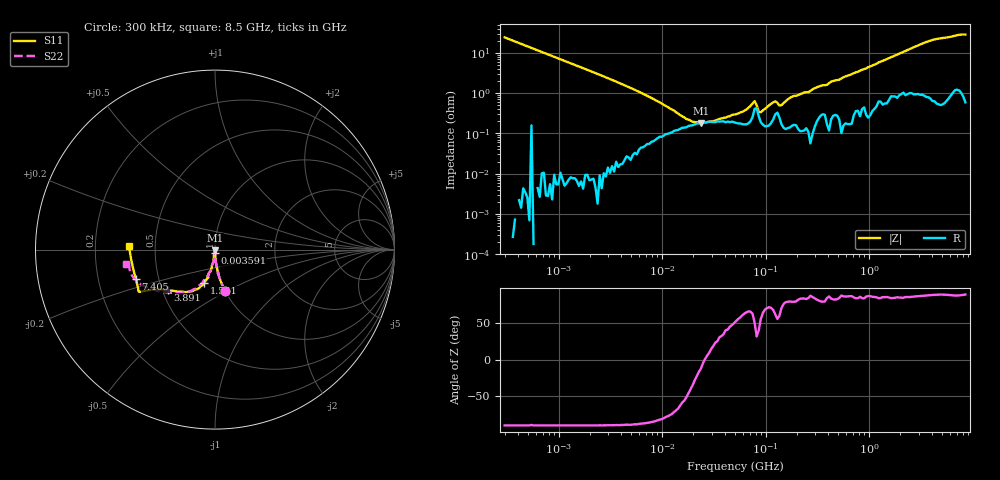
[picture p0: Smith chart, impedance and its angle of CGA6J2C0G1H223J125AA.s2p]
! S-parameter Generated by TDK Corporation
! Copyright(C) 2015 TDK Corporation.
! All Rights Reserved.
! TDK P/N: CGA6J2C0G1H223J125AA (Multilayer Ceramic Chip Capacitors)
! Property: C=22nF
! Size(LxWxT): 3.2x2.5x1.25mm, 0.126x0.098x0.049inches
! Model Type: s2p (Touchstone File Format Version 1.0)
! Frequency: DC=Yes Start=0.3MHz Stop=8500MHz 225points Log-sweep
! Note:
! Model Generated on Jun. 23, 2015
! Hash(MD5):
! Port Assignments:
!  1 ---| |--- 2
! Applicable Conditions:
!  Temperature = 25 degC
!  DC Bias Voltage = 0 V
!  Small Signal Operation
! Terms and conditions regarding TDK Simulation Models
! (1)This simulation model is being provided solely for informational purposes. Please refer to the specifications of the products in terms of detailed characteristics of such products.
! (2)In no event shall TDK Corporation of any of its subsidiaries be liable for any loss or damage arising, directly or indirectly,
!  From any information contained in this simulation model, including, but not limited to loss or damages arising from any inaccuracies, omissions or errors in connection with such information.
! (3)Any and all copyrights on this simulation model are owned by TDK Corporation.
!  Duplication or redistribution of this simulation model without prior written permission from TDK Corporation is prohibited.
! (4)This simulation model is subject to any modification or change without any prior notice.
! (5)Neither TDK Corporation nor any of its subsidiaries shall make any warranty, express or implied,
!  Including but not limited to the correctness, implied warranties of merchantability and fitness for a particular purpose with respect to this simulation models.
! (6)The use of this simulation model shall be deemed to have consented to the terms and conditions hereof.
# MHz S MA R 50
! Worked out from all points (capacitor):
!   224 points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, 300 kHz to 8.5 GHz, reference 50 ohm
!   read as one part in series: C = 22 nF near 314.1 kHz
!   lowest |Z| = 179 mohm at 23.65 MHz (marker M1)
!   series resonance near 25.8 MHz, so ESL is about 1.7 nH
!   S11 on the Smith chart (normalised r, x): 300 kHz: 1.00, -0.48; 3.591 MHz: 1.00, -0.04; 1.551 GHz: 0.83, -0.32; 3.891 GHz: 0.54, -0.27; 7.405 GHz: 0.37, -0.16; 8.5 GHz: 0.35, +0.02
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0.3  0.2356 -76.4  0.9718 13.6  0.9719 13.6  0.2356 -76.5
0.5453461  0.1286 -81.5  0.9894 7.5  0.9869 7.8  0.1318 -83.8
1.72111  0.04191 -87.7  0.9991 2.4  0.999 2.4  0.04189 -87.6
3.591337  0.01996 -88.8  0.9997 1.1  0.9993 1.1  0.01996 -88.5
9.430415  0.007485 -86.8  0.9991 0.2  0.9989 0.2  0.007871 -82.5
14.93432  0.005011 -83.0  0.9986 -0.0  0.9985 -0.0  0.006053 -73.9
23.65048  0.003977 -81.2  0.9983 -0.2  0.9977 -0.2  0.006263 -68.6
34.1636  0.004056 -86.8  0.9975 -0.4  0.9973 -0.4  0.007563 -71.1
51.67171  0.005391 -98.7  0.997 -0.7  0.9968 -0.7  0.01001 -79.6
74.64084  0.007078 -98.0  0.9953 -1.1  0.9952 -1.1  0.01185 -83.1
85.6787  0.01201 -95.8  0.9949 -1.1  0.9947 -1.1  0.01632 -86.4
118.2037  0.01547 -95.3  0.9947 -1.6  0.9945 -1.6  0.01782 -93.3
135.6836  0.02108 -93.5  0.9947 -1.7  0.9943 -1.7  0.02062 -91.9
187.1913  0.0251 -98.8  0.9947 -2.5  0.9945 -2.5  0.02745 -94.2
283.1228  0.04067 -99.9  0.9934 -3.6  0.9931 -3.6  0.0369 -99.4
514.6664  0.07195 -97.8  0.9913 -6.7  0.991 -6.7  0.07509 -98.4
1551.304  0.1951 -107.8  0.9696 -19.8  0.9694 -19.7  0.1866 -110.5
2693.286  0.2798 -123.0  0.9393 -33.4  0.9391 -33.4  0.2817 -123.1
3890.506  0.3459 -139.4  0.9104 -46.9  0.91 -46.9  0.3471 -136.2
5884.306  0.4802 -150.6  0.8511 -66.6  0.8507 -66.6  0.4798 -160.9
7404.957  0.4704 -159.5  0.8329 -78.7  0.8327 -78.6  0.48 -172.3
8500  0.4803 177.4  0.8167 -88.5  0.8173 -88.5  0.503 -171.0
